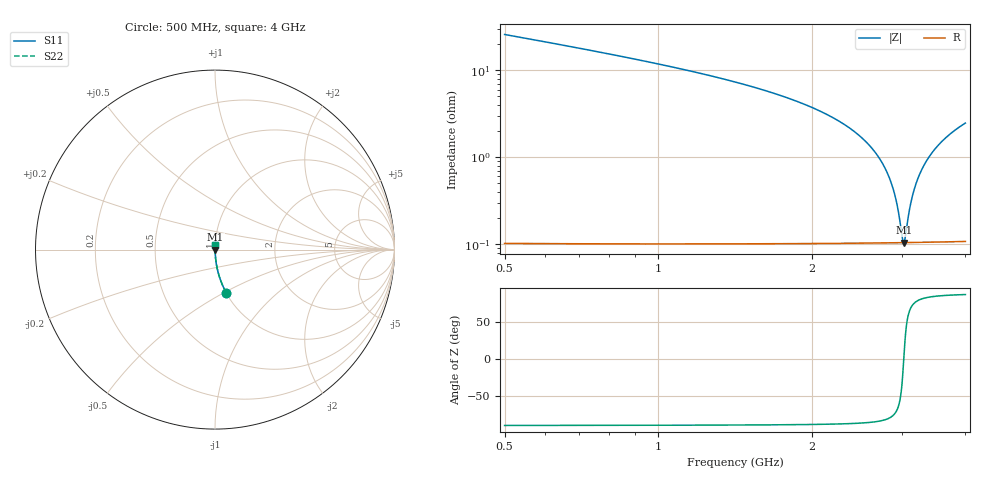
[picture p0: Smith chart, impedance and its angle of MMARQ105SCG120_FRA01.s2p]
! MMARQ105SCG120_FRA01  S-PARAMETER MODEL  ( General Type )
! Model Generated by TAIYO YUDEN Corporation (http://www.ty-top.com)
! Version 1.0
! TAIYO YUDEN Control No. 200326
! Copyright(c) 2020 TAIYO YUDEN CO.,LTD. All Rights Reserved.
! Product Description (link to TY-COMPAS)
! https://ds.yuden.co.jp/TYCOMPAS/or/detail?pn=MMARQ105SCG120JFRA01&u=M
! Products Name : Multilayer Ceramic Capacitors
! Characteristics :
!  Capacitance : 12 pF , Rated Voltage : 250V , TCC : CG / C0G
!  Case Size : 1.0 x 0.5 / 0.039 x 0.02 [mm/inch] , Thickness : 0.5 / 0.02 [mm/inch]
!  (Conditions: Temperature = 25 degC , DC Bias Current/Voltage = 0A / 0V)
! External Node Assignments :
!  1  o---| |---o  2
! GND o---------o GND
! Frequency Range : 500MHz  -  4GHz  [ 401 STEP ]
# MHz S RI R 50
! Freq[MHz].  S11 Real  S11 Imag  S21 Real  S21 Imag  S12 Real  S12 Imag  S22 Real  S22 Imag
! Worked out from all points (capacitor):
!   401 points, 500 MHz to 4 GHz, reference 50 ohm
!   read as one part in series: C = 12 pF near 517.5 MHz
!   lowest |Z| = 104 mohm at 3.029 GHz (marker M1)
!   series resonance near 3.029 GHz, so ESL is about 230 pH
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500  0.0632 -0.2414  0.9368 0.2414  0.9368 0.2414  0.0632 -0.2414
762.5  0.0268 -0.1583  0.9732 0.1583  0.9732 0.1583  0.0268 -0.1583
1086.25  0.0122 -0.105  0.9878 0.105  0.9878 0.105  0.0122 -0.105
1672.5  0.00403 -0.0548  0.996 0.0548  0.996 0.0548  0.00403 -0.0548
2250  0.00171 -0.0263  0.9983 0.0263  0.9983 0.0263  0.00171 -0.0263
2451.25  0.00137 -0.0186  0.9986 0.0186  0.9986 0.0186  0.00137 -0.0186
2608.75  0.0012 -0.0131  0.9988 0.0131  0.9988 0.0131  0.0012 -0.0131
2740  0.00111 -0.00877  0.9989 0.00877  0.9989 0.00877  0.00111 -0.00877
2836.25  0.00107 -0.00574  0.9989 0.00574  0.9989 0.00574  0.00107 -0.00574
2880  0.00105 -0.0044  0.9989 0.0044  0.9989 0.0044  0.00105 -0.0044
2923.75  0.00105 -0.00308  0.999 0.00308  0.999 0.00308  0.00105 -0.00308
2958.75  0.00104 -0.00204  0.999 0.00204  0.999 0.00204  0.00104 -0.00204
3011.25  0.00104 -0.000506  0.999 0.000506  0.999 0.000506  0.00104 -0.000506
3028.75  0.00104 5.93e-07  0.999 -5.93e-07  0.999 -5.93e-07  0.00104 5.93e-07
3046.25  0.00104 0.000504  0.999 -0.000504  0.999 -0.000504  0.00104 0.000504
3098.75  0.00104 0.002  0.999 -0.002  0.999 -0.002  0.00104 0.002
3125  0.00105 0.00273  0.999 -0.00273  0.999 -0.00273  0.00105 0.00273
3186.25  0.00106 0.00443  0.9989 -0.00443  0.9989 -0.00443  0.00106 0.00443
3291.25  0.0011 0.00727  0.9989 -0.00727  0.9989 -0.00727  0.0011 0.00727
3422.5  0.00117 0.0107  0.9988 -0.0107  0.9988 -0.0107  0.00117 0.0107
3667.5  0.00134 0.0168  0.9987 -0.0168  0.9987 -0.0168  0.00134 0.0168
4000  0.00168 0.0246  0.9983 -0.0246  0.9983 -0.0246  0.00168 0.0246
